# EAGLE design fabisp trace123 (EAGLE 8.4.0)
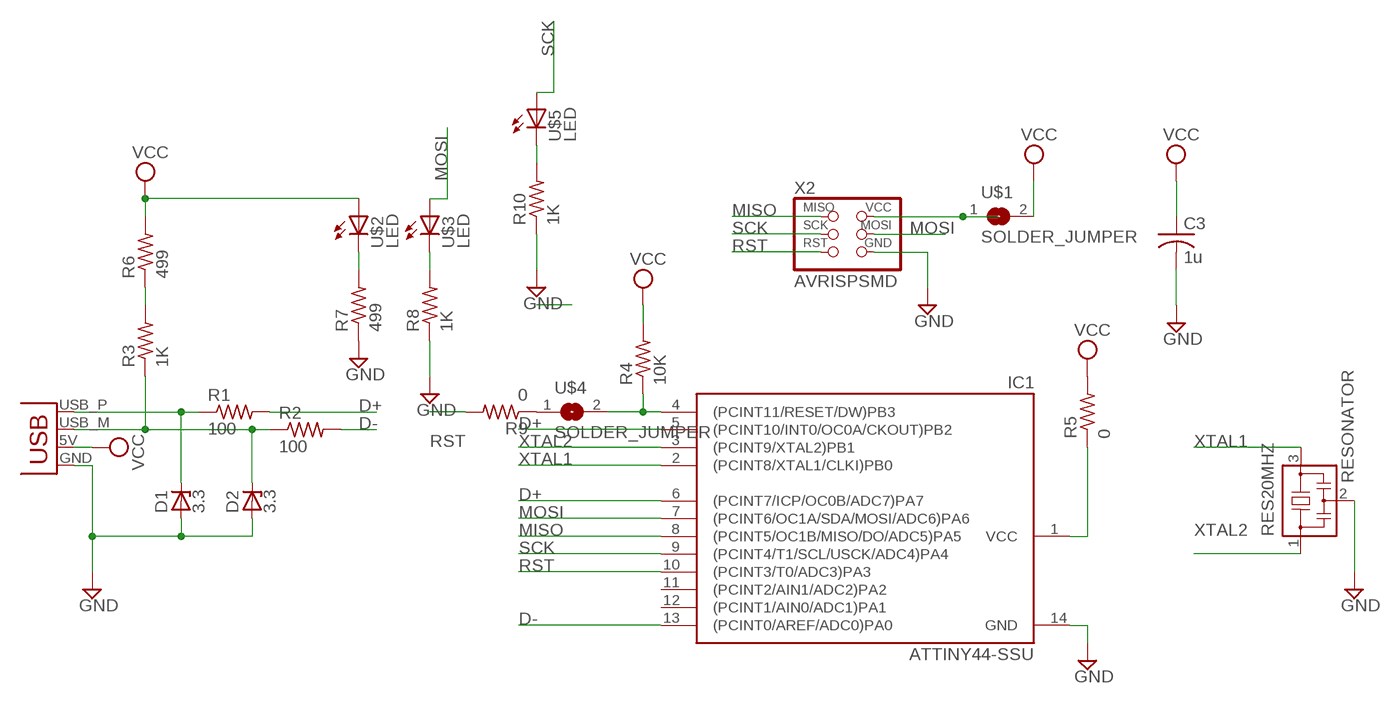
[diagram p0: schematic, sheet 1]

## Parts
C3  1u  C-USC1206  [C1206]
D1  3.3  ZENER_DIODESOD123  [SOD123]
D2  3.3  ZENER_DIODESOD123  [SOD123]
IC1  ATTINY44-SSU  [SOIC14]
R1  100  R-US_R1206  [R1206]
R2  100  R-US_R1206  [R1206]
R3  1K  R-US_R1206  [R1206]
R4  10K  R-US_R1206  [R1206]
R5  0  R-US_R1206  [R1206]
R6  499  R-US_R1206  [R1206]
R7  499  R-US_R1206  [R1206]
R8  1K  R-US_R1206  [R1206]
R9  0  R-US_R1206  [R1206]
R10  1K  R-US_R1206  [R1206]
RES20MHZ  RESONATOR  [EFOBM]
U$1  SOLDER_JUMPER  [SJFAB]
U$2  LED  [LED1206]
U$3  LED  [LED1206]
U$4  SOLDER_JUMPER  [SJFAB]
U$5  LED  [LED1206]
X1  USBPCB  [USB-A-PCB]
X2  AVRISPSMD  [2X03SMD]

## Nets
D+: IC1.5((PCINT10/INT0/OC0A/CKOUT)PB2) IC1.6((PCINT7/ICP/OC0B/ADC7)PA7) R1.2
D-: IC1.13((PCINT0/AREF/ADC0)PA0) R2.2
GND: C3.2 D1.ANODE D2.ANODE IC1.14(GND) R7.1 R8.1 R10.1 RES20MHZ.2 X1.GND X2.6(GND)
MISO: IC1.8((PCINT5/OC1B/MISO/DO/ADC5)PA5) X2.1(MISO)
MOSI: IC1.7((PCINT6/OC1A/SDA/MOSI/ADC6)PA6) U$3.1(A) X2.4(MOSI)
N$1: D1.CATHODE R1.1 X1.USB_P(D+)
N$2: D2.CATHODE R2.1 R3.1 X1.USB_M(D-)
N$3: IC1.4((PCINT11/RESET/DW)PB3) R4.1 U$4.2
N$4: R7.2 U$2.2(C)
N$5: R8.2 U$3.2(C)
N$6: R3.2 R6.1
N$7: U$1.1 X2.2(VCC)
N$8: R10.2 U$5.2(C)
N$9: IC1.1(VCC) R5.1
N$10: R9.1 U$4.1
RST: IC1.10((PCINT3/T0/ADC3)PA3) R9.2 X2.5(RST)
SCK: IC1.9((PCINT4/T1/SCL/USCK/ADC4)PA4) U$5.1(A) X2.3(SCK)
VCC: C3.1 R4.2 R5.2 R6.2 U$1.2 U$2.1(A) X1.5V(VBUS)
XTAL1: IC1.2((PCINT8/XTAL1/CLKI)PB0) RES20MHZ.3
XTAL2: IC1.3((PCINT9/XTAL2)PB1) RES20MHZ.1
Unconnected: IC1.11((PCINT2/AIN1/ADC2)PA2) IC1.12((PCINT1/AIN0/ADC1)PA1)

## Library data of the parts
C3 = rcl:C-US: CAPACITOR, American symbol
D1 D2 = fab:ZENER_DIODE: zener diode
IC1 = fab:ATTINY44
R1-R10 = rcl:R-US_: RESISTOR, American symbol
RES20MHZ = fab:RESONATOR
U$1 U$4 = fab:SOLDER_JUMPER
U$2 U$3 U$5 = fab:LED: LED
X1 = SparkFun:USB: USB Connectors USB-B-PTH is fully proven SKU : PRT-00139 USB-miniB is fully proven SKU : PRT-00587 USB-A-PCB is untested. USB-A-H is throughly reviewed, but untested. Spark Fun Electronics SKU : PRT-00437 USB-B-SMT is throughly reviewed, but untested. Needs silkscreen touching up. USB-A-S has not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
X2 = fab:AVRISP

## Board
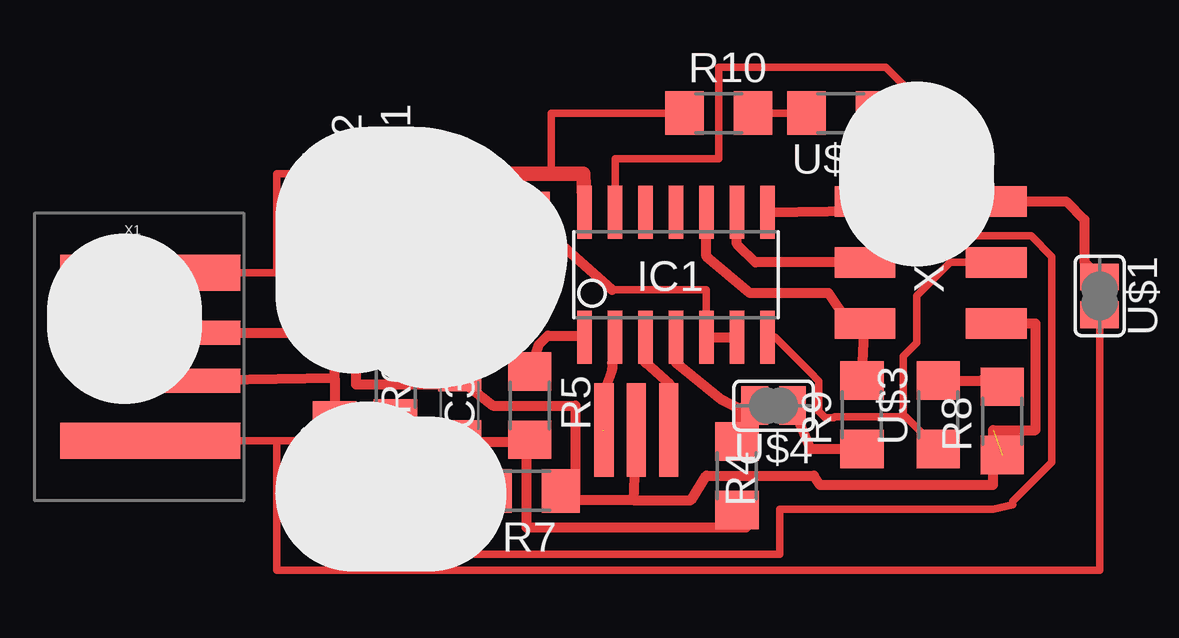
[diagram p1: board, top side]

No outline drawn. Coordinates in mm, seen from the top.
Copper layers (1*16): Top 0.035mm / dielectric 1.5mm / Bottom 0.035mm
Design rules "fab": minimum track width 12mil, minimum drill 0.8mm, track to track 15.5mil, track to pad 15.5mil, pad to pad 15mil, via to via 15mil, smd to smd 10mil, copper to edge 0mil, drill to drill 1mm, minimum pad ring 0.2mm, minimum via ring 0.2mm, stop-mask expansion 4mil, vias tented up to drill 0mil, thermal gap 1mm

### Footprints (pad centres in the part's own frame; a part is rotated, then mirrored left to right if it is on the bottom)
C1206 = smd 1.6 x 1.8: 1 -1.4,0; 2 1.4,0
SOD123 = smd 1.6 x 0.8: ANODE 1.7,0; CATHODE -1.7,0
SOIC14 = smd 0.61 x 2.21: 1 -3.81,-2.603; 2 -2.54,-2.603; 3 -1.27,-2.603; 4 0,-2.603; 5 1.27,-2.603; 6 2.54,-2.603; 7 3.81,-2.603; 8 3.81,2.603; 9 2.54,2.603; 10 1.27,2.603; 11 0,2.603; 12 -1.27,2.603; 13 -2.54,2.603; 14 -3.81,2.603
R1206 = smd 1.6 x 1.803: 1 -1.422,0; 2 1.422,0
EFOBM = smd 0.8 x 3.9: 1 -1.35,0; 2 0,0; 3 1.35,0
SJFAB = smd 1.118 x 1.6: 1 -0.787,0; 2 0.787,0
LED1206 = smd 1.6 x 1.803: 1 -1.422,0; 2 1.422,0
USB-A-PCB = smd 7.5 x 1.5: 5V -0.2,-3.5; GND -0.2,3.5 | smd 6.5 x 1: USB_M 0.3,-1; USB_P 0.3,1
2X03SMD = smd 2.54 x 1.27: 1 -2.54,2.54; 2 2.92,2.54; 3 -2.54,0; 4 2.92,0; 5 -2.54,-2.54; 6 2.92,-2.54

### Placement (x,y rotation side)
C3  17.78,6.22 90 top
D1  15.11,14.1 90 top
D2  13.08,13.59 90 top
IC1  26.8,11.68 0 top
R1  19.3,14.22 0 top
R2  12.57,4.19 270 top
R3  19.3,11.56 0 top
R4  29.34,3.3 270 top
R5  20.7,6.22 270 top
R6  15.11,7.11 270 top
R7  20.57,2.67 180 top
R8  40.39,5.59 90 top
R9  34.54,5.84 90 top
R10  28.57,18.41 0 top
RES20MHZ  25.15,5.21 180 top
U$1  44.45,10.79 270 top
U$2  16.13,2.67 0 top
U$3  37.72,5.84 90 top
U$4  30.86,6.22 180 top
U$5  33.66,18.41 180 top
X1  5.08,8.26 0 top
X2  37.21,12.19 0 top

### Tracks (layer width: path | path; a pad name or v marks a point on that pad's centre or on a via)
D+
  Top 0.305: 24.13,11.05 28.07,11.05 IC1.5
  Top 0.406: IC1.5 IC1.6 | 24.13,11.05 21.87,13.08 R1.2
D-
  Top 0.152: R2.2 12.7,2.64 | 40.83,2.1 40.83,2.25
  Top 0.305: 12.7,2.64 12.7,1.03 17.42,1.03 18.41,0.04 31.11,0.04 31.11,1.91 40.01,1.91 40.83,2.1 | 40.83,2.25 42.46,3.87 42.46,12.44 41.6,13.3 38.67,13.3 37.45,15.12 37.45,18.41 35.54,20.32 28.57,20.32 28.57,16.51 24.26,16.51 IC1.13
GND  (1 unrouted)
  Top 0.152: 13.2,15.88 13.2,15.75
  Top 0.305: R10.1 21.59,18.41 21.59,15.88 | X1.GND 10.16,11.76 10.16,15.88 13.2,15.88
  Top 0.406: 40.13,9.4 X2.6 41.78,9.65 41.78,5.21 40.01,5.21 40.01,2.92 32.8,2.92 32.54,3.3 28.07,3.3 27.43,2.29 25.02,2.29 | RES20MHZ.2 25.02,2.29 | 19.3,15.88 19.3,10.54 19.05,10.03 13.46,10.03 13.46,7.11 17.78,7.11 | 17.78,7.11 C3.2 | D2.ANODE 13.2,15.75 13.21,15.8 | 25.02,2.29 22.61,2.29 | 22.61,2.29 21.87,2.67 R7.1 | 22.61,2.29 22.61,6.22 19.18,6.22 18.03,7.11 17.78,7.11
  Top 0.61: 13.21,15.8 D1.ANODE 19.3,15.88 21.59,15.88 22.92,15.88 IC1.14
MISO
  Top 0.406: IC1.8 34.42,14.35 X2.1
MOSI
  Top 0.305: IC1.7 30.92,9.08 32.38,7.62 32.75,7.25 32.75,5.98 33.02,5.71 33.37,5.71 33.42,5.77 36.2,5.77 | 36.2,5.77 36.37,5.77 U$3.1 | X2.4 38.23,12.19 36.83,10.79 36.83,8.85 36.27,8.29 36.27,5.84 36.2,5.77
N$1
  Top 0.406: X1.USB_P 11.72,9.26 11.68,12.52 12.32,13.72 14.86,13.72 14.78,12.27 D1.CATHODE 17.19,14.22 R1.1
N$2
  Top 0.406: 12.57,7.37 5.4,7.24 X1.USB_M | 12.57,7.37 R2.1 | 12.57,7.37 12.57,11 D2.CATHODE 12.62,10.87 17.27,10.92 R3.1
N$3
  Top 0.406: IC1.4 26.8,8 28.7,6.48 | 28.7,6.48 29.46,6.12 R4.1 | U$4.2 29.36,6.12 28.7,6.48
N$4
  Top 0.406: U$2.2 R7.2
N$5
  Top 0.406: U$3.2 39.5,7.26 R8.2
N$6
  Top 0.406: R6.1 15.04,9.17 19.46,9.17 20.7,10.16 R3.2
N$7
  Top 0.406: X2.2 43.05,14.73 43.81,13.97 43.81,12.22 U$1.1
N$8
  Top 0.305: R10.2 U$5.2
N$9
  Top 0.406: R5.1 21.08,8.76 21.46,9.14 22.92,9.14 IC1.1
N$10
  Top 0.406: U$4.1 32.38,4.42 R9.1
RST
  Top 0.406: IC1.10 28.07,12.45 29.87,10.92 33.15,10.92 33.91,9.78 X2.5 R9.2
SCK
  Top 0.305: 35.08,17.63 U$5.1 35.56,17.78 36.83,16.51 36.83,13.34 35.56,12.06 34.8,12.06 X2.3
  Top 0.406: IC1.9 29.34,12.95 30.1,12.19 X2.3
VCC
  Top 0.152: R6.2 14.71,5.69 | 14.71,3.31 U$2.1
  Top 0.305: U$2.1 14.71,5.69 | 10.16,4.75 X1.5V | 10.16,4.75 11.06,4.75 11.48,4.34 13.67,4.34 14.71,3.31 | U$1.2 44.45,-0.64 10.16,-0.64 10.16,4.75
  Top 0.406: 29.72,2.03 29.72,1.14 29.46,1.14 | 29.46,1.14 20.57,1.14 20.57,4.7 | R4.2 29.46,1.14 | R6.2 16.11,4.82 C3.1 17.78,4.7 20.57,4.7 | R5.2 20.55,4.67 20.57,4.7
XTAL1  (1 unrouted)
  Top 0.406: IC1.2 24.26,8.13 24.13,8 24.13,7.75 23.88,6.99 23.62,5.21 23.75,5.21
XTAL2
  Top 0.406: IC1.3 25.53,8 26.54,7.11 26.54,6.05 RES20MHZ.1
